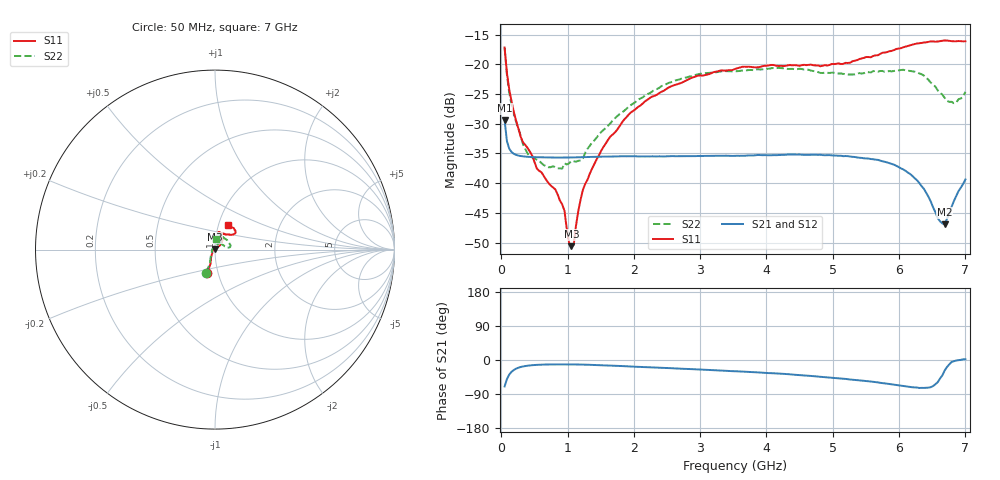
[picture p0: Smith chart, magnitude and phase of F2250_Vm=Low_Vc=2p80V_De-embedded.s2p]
! Integrated Device Technology
! Corporate Headquarters
! 6024 Silver Creek Valley Road
! San Jose, CA 95138  USA
! Phone:  1-408-284-8200
! Toll Free:  1-800-223-1366
! Webpage:  http://www.idt.com/
! Timing and RF Division
! 515 Groton Road, Suite 102
! Westford, MA 01886-6024
! Device:  F2250
! Description: Voltage Variable RF Attenuator
! Frequency:  50.0 -  6000.00 MHz
! Package:  3x3 mm Thin QFN Plastic Package: 16 pin
! Ports:  2 RF, 3 DC
!  Pin  1  = GND
!  Pin  2  = NC
!  Pin  3  = RF1  = Port 1
!  Pin  4  = NC
!  Pin  5  = GND
!  Pin  6  = GND
!  Pin  7  = GND
!  Pin  8  = GND
!  Pin  9  = NC
!  Pin 10  = RF2  = Port 2
!  Pin 11  = NC
!  Pin 12  = GND
!  Pin 13  = GND
!  Pin 14  = VCNTRL
!  Pin 15  = VDD
!  Pin 16  = VMODE
! Vcntrl:  2.800 Volts
! Vmode:  +0.000 Volts
! Vdd:  +3.30  Volts
! Current:  1.177 mA
! Data:  The device was measured on a the F2250 evaluation board which has
!  individual transmission lines to the RF pins.  Data was collected
!  using a calibrated network analyzer.  The evaluation board was
!  de-embedded using a TRL calibration technique.
!  The reference plane is the edge of the package pin.
! Misc:  SN 10
!  Action Tracker AT0258
! Date Measured:  2014-11-26
! Date:  2015-10-15  MJV
! Note:
!  Integrated Device Technology supplies this data as a sample of measured
!  data at the package pin for this product.  Your particular data for this
!  product may vary.
!  Data was taken at 25 degrees C.
!  Integrated Device Technology reserves the right to change this data at anytime.
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# GHz S dB R 50
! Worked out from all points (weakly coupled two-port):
!   201 points, 50 MHz to 7 GHz, reference 50 ohm
!   highest |S21| = -29.41 dB at 50 MHz (marker M1); lowest = -46.9 dB at 6.687 GHz (marker M2)
!   lowest |S11| = -50.6 dB at 1.058 GHz (marker M3), VSWR 1.01, Z = 49.8 + j0.247 ohm
!   |S11| at or under -10 dB: start of sweep to end of sweep
!   |S22| runs from -37.5 to -17.3 dB; largest |S21 - S12| = 7.2e-05
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0.05  -17.18 -108.7  -29.41 -69.8  -29.41 -69.8  -17.27 -111.0
0.08475  -21.45 -107.5  -32.92 -50.3  -32.92 -50.4  -21.75 -110.2
0.15425  -26.22 -116.6  -34.76 -31.2  -34.76 -31.2  -26.82 -122.4
0.29325  -32.21 -127.8  -35.43 -18.5  -35.43 -18.5  -32.10 -137.4
0.3975  -34.09 -141.8  -35.56 -15.0  -35.56 -15.0  -35.03 -160.4
0.91875  -43.55 157.6  -35.68 -11.5  -35.68 -11.5  -37.53 133.4
0.9535  -44.66 170.0  -35.69 -11.5  -35.68 -11.5  -36.66 131.0
1.023  -50.03 143.7  -35.68 -11.6  -35.67 -11.6  -36.64 115.9
1.05775  -50.59 122.9  -35.67 -11.6  -35.67 -11.6  -36.27 110.7
1.0925  -50.37 90.6  -35.66 -11.7  -35.66 -11.7  -36.31 106.5
1.162  -44.66 57.1  -35.64 -11.9  -35.64 -11.9  -36.22 95.5
1.2315  -41.09 44.2  -35.61 -12.1  -35.61 -12.1  -35.81 85.8
1.6485  -32.11 41.9  -35.52 -14.6  -35.52 -14.6  -29.88 64.5
1.96125  -28.04 42.1  -35.46 -17.2  -35.46 -17.2  -26.81 56.8
2.37825  -24.87 47.3  -35.48 -20.3  -35.48 -20.3  -23.99 56.8
3.525  -20.79 72.5  -35.40 -29.5  -35.40 -29.5  -21.19 74.7
4.7065  -20.17 72.4  -35.20 -42.6  -35.20 -42.6  -21.14 72.3
5.85325  -17.82 40.5  -36.63 -63.3  -36.64 -63.4  -21.14 23.1
6.27025  -16.51 40.0  -39.50 -72.7  -39.51 -72.8  -21.36 9.7
6.68725  -15.99 48.8  -46.88 -27.7  -46.86 -27.4  -25.64 28.5
6.861  -16.13 55.1  -42.19 -1.3  -42.14 -1.3  -26.46 57.9
7  -16.13 63.2  -39.37 1.9  -39.31 1.7  -24.63 83.1
